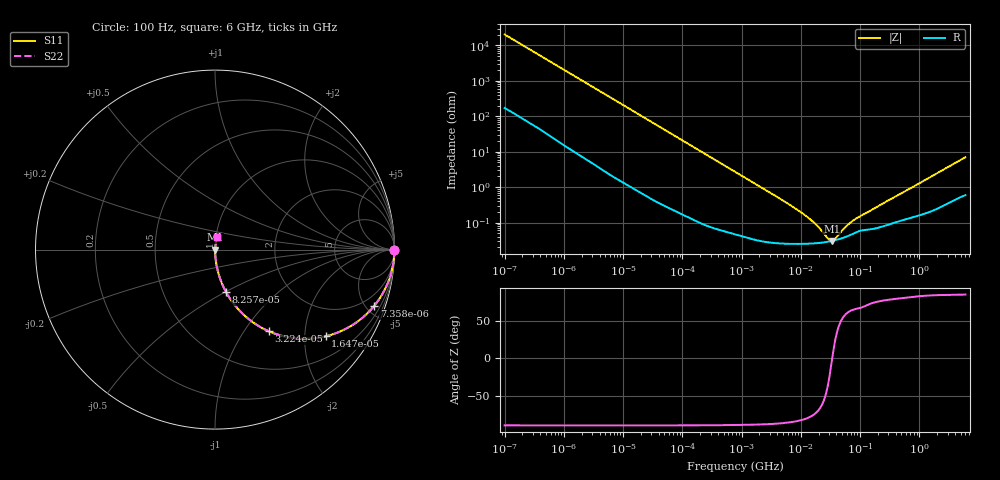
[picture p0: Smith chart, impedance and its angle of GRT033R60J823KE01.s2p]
!Murata Part Number: GRT033R60J823KE01
!These Parameters are Measured in Series Mode Connection
!Data Generated on Jun 19, 2026
!  o--ll--o
!Port1  Port2
!  o------o
!Operation Temp=25[degC], DC Bias Voltage=0[V]
!Freq. Start=100[Hz] Stop=6[GHz] 401[Steps]
# Hz S RI R 50
!Freq.(Hz) S11(Real) S11(Imag) S21(Real) S21(Imag) S12(Real) S12(Imag) S22(Real) S22(Imag)
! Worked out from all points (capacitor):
!   401 points, 100 Hz to 6 GHz, reference 50 ohm
!   read as one part in series: C = 77.8 nF near 109 Hz
!   lowest |Z| = 30.3 mohm at 33.3 MHz (marker M1)
!   series resonance near 33.9 MHz, so ESL is about 280 pH
!   S11 on the Smith chart (normalised r, x): 100 Hz: open; 7.358 kHz: 1.04, -5.66; 16.47 kHz: 1.02, -2.54; 32.24 kHz: 1.01, -1.30; 82.57 kHz: 1.00, -0.51; 6 GHz: 1.01, +0.14
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100  0.9999 -0.0049  6.53e-05 0.0049  6.53e-05 0.0049  0.9999 -0.0049
627  0.9988 -0.0304  0.00116 0.0304  0.00116 0.0304  0.9988 -0.0304
2008  0.99 -0.0959  0.00997 0.0959  0.00997 0.0959  0.99 -0.0959
4299  0.9578 -0.1978  0.0422 0.1978  0.0422 0.1978  0.9578 -0.1978
7358  0.8875 -0.3127  0.1125 0.3127  0.1125 0.3127  0.8875 -0.3127
11009  0.7807 -0.4105  0.2193 0.4105  0.2193 0.4105  0.7807 -0.4105
16473  0.6161 -0.483  0.3839 0.483  0.3839 0.483  0.6161 -0.483
22537  0.4633 -0.4954  0.5367 0.4954  0.5367 0.4954  0.4633 -0.4954
32244  0.2982 -0.4542  0.7018 0.4542  0.7018 0.4542  0.2982 -0.4542
40335  0.2144 -0.407  0.7856 0.407  0.7856 0.407  0.2144 -0.407
82567  0.0626 -0.2383  0.9374 0.2383  0.9374 0.2383  0.0626 -0.2383
221108  0.00993 -0.0945  0.9901 0.0945  0.9901 0.0945  0.00993 -0.0945
774597  0.00122 -0.0274  0.9988 0.0274  0.9988 0.0274  0.00122 -0.0274
6353432  0.000262 -0.00325  0.9997 0.00325  0.9997 0.00325  0.000262 -0.00325
1.555665e7  0.000258 -0.00108  0.9997 0.00108  0.9997 0.00108  0.000258 -0.00108
2.911731e7  0.000289 -0.000189  0.9997 0.000189  0.9997 0.000189  0.000289 -0.000189
3.330331e7  0.000302 -2.14e-05  0.9997 2.14e-05  0.9997 2.14e-05  0.000302 -2.14e-05
3.80911e7  0.000318 0.000143  0.9997 -0.000143  0.9997 -0.000143  0.000318 0.000143
5.699437e7  0.000393 0.000645  0.9996 -0.000645  0.9996 -0.000645  0.000393 0.000645
7.797396e7  0.000493 0.00106  0.9995 -0.00106  0.9995 -0.00106  0.000493 0.00106
3.124326e8  0.000908 0.00429  0.9991 -0.00429  0.9991 -0.00429  0.000908 0.00429
6e9  0.0106 0.0683  0.9894 -0.0683  0.9894 -0.0683  0.0106 0.0683
